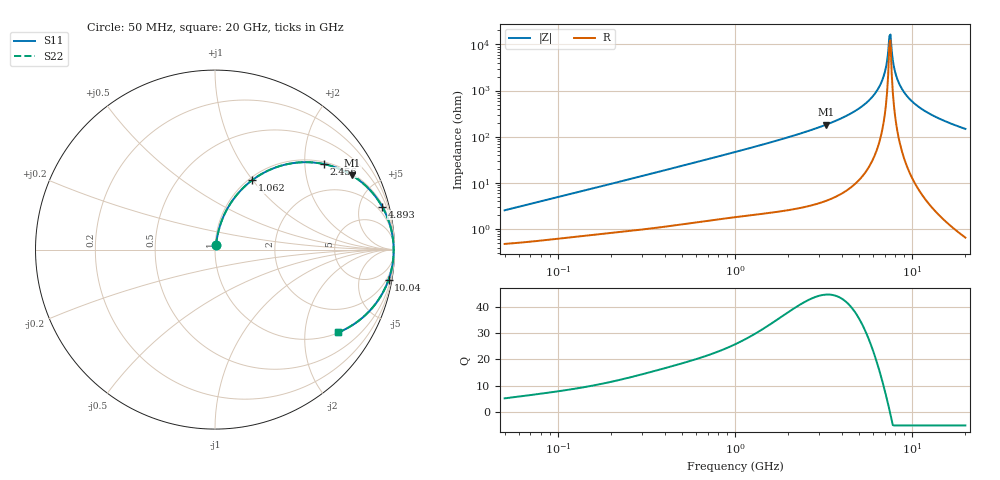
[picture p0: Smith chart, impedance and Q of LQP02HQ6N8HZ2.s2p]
!Murata Part Number: LQP02HQ6N8HZ2
!These Parameters are Measured in Series Mode Connection
!  o--[Z]--o
!Port1  Port2
!  o-------o
!Freq. Start=50[MHz] Stop=20[GHz], 401[Steps]
# Hz S RI R 50
!Freq.(Hz) S11(Real) S11(Imag) S21(Real) S21(Imag) S12(Real) S12(Imag) S22(Real) S22(Imag)
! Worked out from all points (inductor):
!   401 points, 50 MHz to 20 GHz, reference 50 ohm
!   read as one part in series: L = 7.96 nH near 51.52 MHz
!   highest Q = 44.5 at 3.265 GHz (marker M1), where L = 8.9 nH
!   self-resonance near 7.442 GHz
!   S11 on the Smith chart (normalised r, x): 50 MHz: 1.01, +0.05; 1.062 GHz: 1.04, +0.99; 2.456 GHz: 1.06, +2.50; 4.893 GHz: 1.21, +7.70; 10.04 GHz: 1, -11; 20 GHz: 1.01, -2.96
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5e7  0.00541 0.025  0.9946 -0.025  0.9946 -0.025  0.00541 0.025
1.364002e8  0.0113 0.065  0.9887 -0.065  0.9887 -0.065  0.0113 0.065
3.721004e8  0.0397 0.1665  0.9603 -0.1665  0.9603 -0.1665  0.0397 0.1665
1e9  0.1888 0.3723  0.8112 -0.3723  0.8112 -0.3723  0.1888 0.3723
1.061746e9  0.2069 0.3867  0.7931 -0.3867  0.7931 -0.3867  0.2069 0.3867
1.714689e9  0.4069 0.4771  0.5931 -0.4771  0.5931 -0.4771  0.4069 0.4771
2.456456e9  0.6069 0.4766  0.3931 -0.4766  0.3931 -0.4766  0.6069 0.4766
2.728004e9  0.6667 0.4599  0.3333 -0.4599  0.3333 -0.4599  0.6667 0.4599
3.265178e9  0.7642 0.4134  0.2358 -0.4134  0.2358 -0.4134  0.7642 0.4134
4.89267e9  0.9312 0.2399  0.0688 -0.2399  0.0688 -0.2399  0.9312 0.2399
5.769027e9  0.9707 0.151  0.0293 -0.151  0.0293 -0.151  0.9707 0.151
6.503449e9  0.9878 0.083  0.0122 -0.083  0.0122 -0.083  0.9878 0.083
7.009217e9  0.9936 0.0397  0.00642 -0.0397  0.00642 -0.0397  0.9936 0.0397
7.331367e9  0.9952 0.0135  0.00484 -0.0135  0.00484 -0.0135  0.9952 0.0135
7.442007e9  0.9954 0.00474  0.00463 -0.00474  0.00463 -0.00474  0.9954 0.00474
7.668323e9  0.9953 -0.0127  0.00466 0.0127  0.00466 0.0127  0.9953 -0.0127
8.020766e9  0.9941 -0.039  0.00587 0.039  0.00587 0.039  0.9941 -0.039
8.389408e9  0.9915 -0.0651  0.00848 0.0651  0.00848 0.0651  0.9915 -0.0651
9.041845e9  0.9841 -0.1084  0.0159 0.1084  0.0159 0.1084  0.9841 -0.1084
1.004137e10  0.9671 -0.1678  0.0329 0.1678  0.0329 0.1678  0.9671 -0.1678
1.334722e10  0.8839 -0.3158  0.1161 0.3158  0.1161 0.3158  0.8839 -0.3158
2e10  0.6863 -0.4618  0.3137 0.4618  0.3137 0.4618  0.6863 -0.4618
